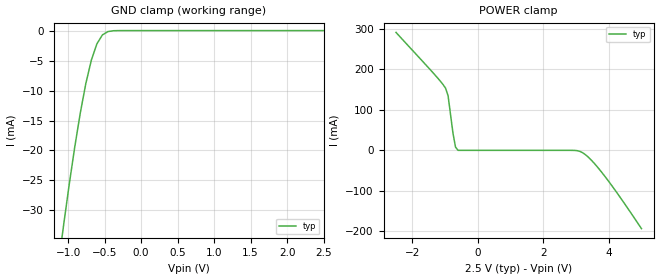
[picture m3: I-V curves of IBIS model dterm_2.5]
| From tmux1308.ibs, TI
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| dterm_2.5
[Model]   dterm_2.5
Model_type   Terminator
|   typ   min   max
C_comp   6.362683e-12   NA   NA
[Voltage Range]   2.5   NA   NA
[Temperature Range]   27   NA   NA
[Power Clamp Reference]   2.5   NA   NA
[GND Clamp Reference]   0   NA   NA
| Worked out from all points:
|   GND clamp passes 1 mA (typ) near -0.54 V on its own axis
|   POWER clamp passes 1 mA (typ) near -0.61 V on its own axis
[GND Clamp]
|   Voltage   I(typ)   I(min)   I(max)
-5V       -20.06kA   NA         NA
-1.136V   -39.38mA   NA         NA
-1.061V   -32.33mA   NA         NA
-909.1mV  -19.41mA   NA         NA
-833.3mV  -13.75mA   NA         NA
-757.6mV  -8.842mA   NA         NA
-681.8mV  -4.933mA   NA         NA
-606.1mV  -2.22mA    NA         NA
-530.3mV  -723.9uA   NA         NA
-454.5mV  -163.6uA   NA         NA
-303mV    -3.411uA   NA         NA
2.5V      1.169nA    NA         NA
[POWER Clamp]
|   Voltage   I(typ)   I(min)   I(max)
-2.5V     290.7mA    NA         NA
-1.288V   183.9mA    NA         NA
-984.9mV  153.1mA    NA         NA
-909.1mV  134.8mA    NA         NA
-757.6mV  41.57mA    NA         NA
-681.8mV  8.261mA    NA         NA
-606.1mV  46.18uA    NA         NA
3.106V    -2.22mA    NA         NA
3.409V    -19.41mA   NA         NA
3.788V    -54.32mA   NA         NA
4.318V    -112.3mA   NA         NA
5V        -193mA     NA         NA
